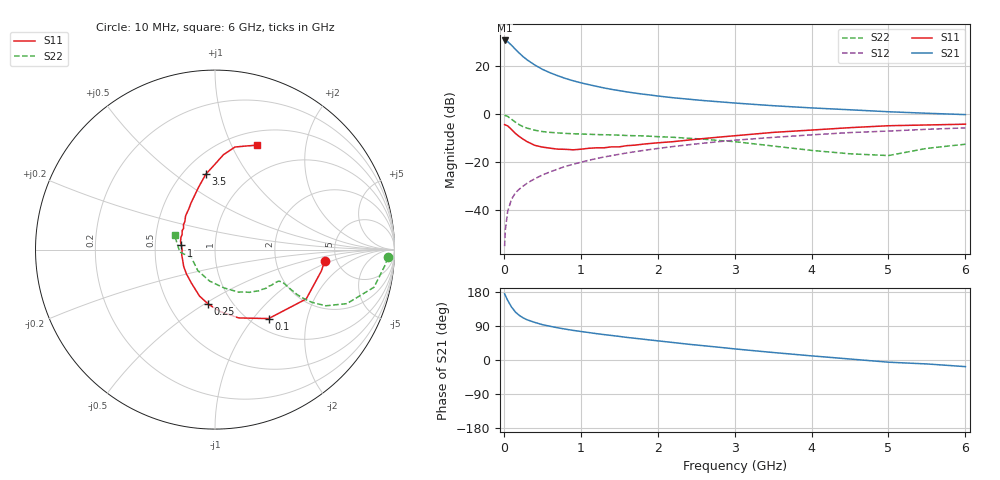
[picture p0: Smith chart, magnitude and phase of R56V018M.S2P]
! SIEMENS Small Signal Semiconductors
! BFR183
! Si NPN RF Bipolar Junction Transistor in SOT23
! VCE = 6 V  IC = 18 mA
! Common Emitter S-Parameters:  May  1996
# GHz  S  MA  R  50
!  f  S11  S21  S12  S22
! GHz  MAG  ANG  MAG  ANG  MAG  ANG  MAG  ANG
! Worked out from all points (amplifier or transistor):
!   36 points, 10 MHz to 6 GHz, reference 50 ohm
!   highest |S21| = 30.8 dB at 10 MHz (marker M1)
!   |S21| within 3 dB of that: start of sweep to 130.1 MHz
!   unconditionally stable (mu >= 1): 623.6 MHz to 2.486 GHz
!   at 250 MHz: K = 0.77, MSG = 27.0 dB, |S12| = -29.9 dB
!   at 1.4 GHz: K = 1.04, MAG = 12.6 dB, |S12| = -17.2 dB
!   at 6 GHz: K = 0.90, MSG = 2.8 dB, |S12| = -5.6 dB
!   S11 on the Smith chart (normalised r, x): 10 MHz: 4.01, -0.82; 100 MHz: 1.19, -1.20; 250 MHz: 0.77, -0.52; 1 GHz: 0.68, +0.03; 3.5 GHz: 0.64, +0.65; 6 GHz: 0.66, +1.26
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0.01  0.6147 -5.9  34.84 174.8  0.0018 83.6  0.9648 -2.6
0.02  0.6046 -11.3  34.41 170.1  0.004 90.9  0.95 -5.5
0.05  0.5779 -28.4  32.82 157.3  0.0096 80.0  0.9106 -13.3
0.1  0.4869 -52.1  27.73 139.8  0.0171 72.0  0.7937 -22.3
0.15  0.4029 -70.9  22.82 126.6  0.0232 67.8  0.6919 -26.9
0.2  0.3469 -85.1  19.03 117.8  0.0277 67.8  0.6124 -28.6
0.25  0.3056 -97.2  16.04 111.3  0.032 67.2  0.5564 -28.9
0.3  0.2727 -108.5  13.83 106.3  0.0367 68.3  0.5204 -28.7
0.4  0.2279 -125.4  10.79 99.3  0.0456 69.0  0.4701 -27.5
0.5  0.2089 -139.6  8.754 93.4  0.0546 69.8  0.4406 -26.5
0.6  0.1985 -151.4  7.403 89.0  0.0636 70.2  0.4238 -26.0
0.7  0.1894 -162.1  6.417 85.0  0.0727 70.4  0.4127 -26.0
0.8  0.1877 -170.8  5.633 81.5  0.0827 69.9  0.4032 -26.1
1  0.1885 173.0  4.577 75.3  0.1008 69.4  0.3917 -27.0
1.1  0.197 167.1  4.197 72.5  0.1107 68.7  0.3865 -28.1
1.3  0.2018 155.3  3.577 67.1  0.1297 67.2  0.3777 -29.9
1.6  0.224 141.7  2.95 59.6  0.1578 64.6  0.3641 -33.8
2.2  0.2711 122.3  2.23 46.1  0.2147 58.5  0.3345 -43.4
3.5  0.4228 97.0  1.522 19.8  0.3329 42.6  0.22 -76.5
4.5  0.531 84.9  1.251 2.6  0.4191 30.3  0.1514 -129.2
5.5  0.6039 73.0  1.059 -10.4  0.4905 18.8  0.1968 -176.0
6  0.6268 68.1  0.993 -17.5  0.5251 11.3  0.2396 160.2
